(* Logix 5000 AddOnInstructionDefinition export Banner_IC70_Param_v4; software revision 33.03; part 2 of 2 *)
(* tags used below, declared in another part *)
   Hub : Banner_IC70_16P_v4;
   Port_Data : Banner_IOL_Port_v4;
   Port : INT;
   Control : DINT;
   Command_Being_Processed : BOOL;
   Index_Write_Inprocess : INT;
   Inprocess_Index : DINT;
   Index5 : SINT;
(* Banner_IC70_Param_v4, continued *)

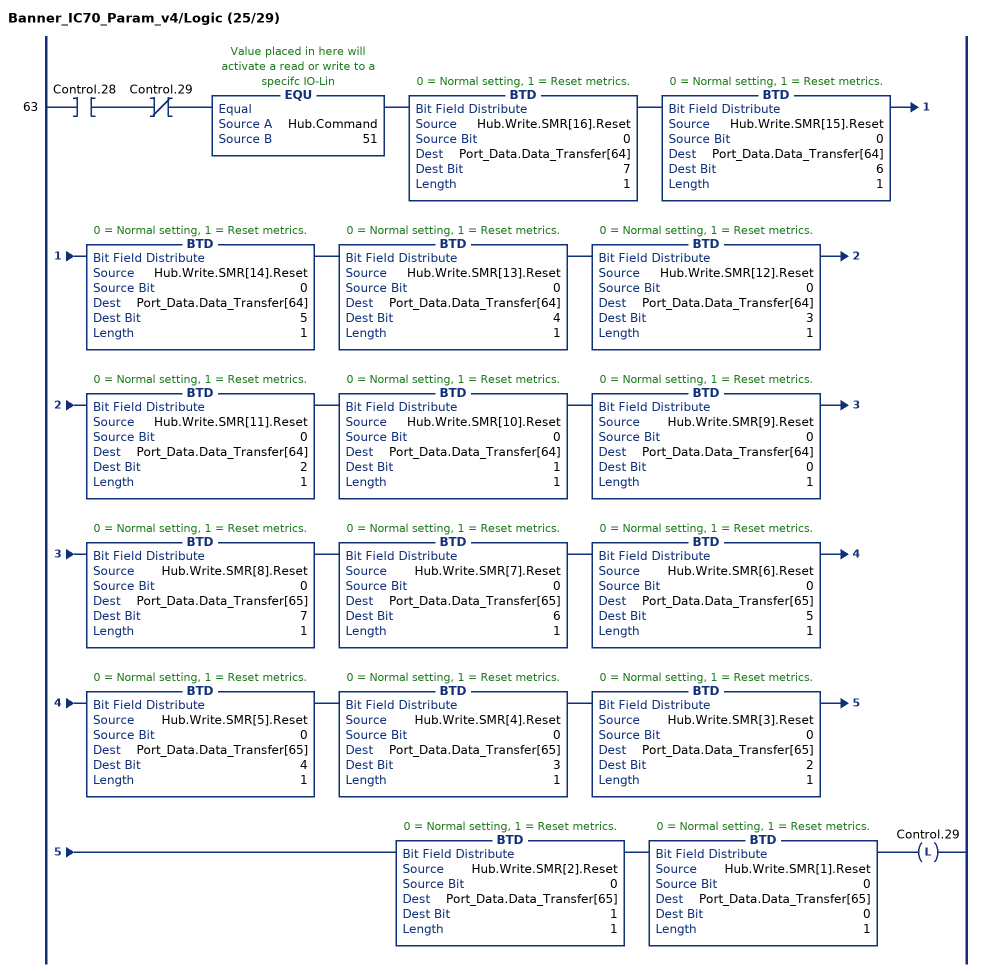
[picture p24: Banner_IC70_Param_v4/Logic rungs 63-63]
   63: XIC(Control.28)XIO(Control.29)EQU(Hub.Command,51)BTD(Hub.Write.SMR[16].Reset,0,Port_Data.Data_Transfer[64],7,1)BTD(Hub.Write.SMR[15].Reset,0,Port_Data.Data_Transfer[64],6,1)BTD(Hub.Write.SMR[14].Reset,0,Port_Data.Data_Transfer[64],5,1)BTD(Hub.Write.SMR[13].Reset,0,Port_Data.Data_Transfer[64],4,1)BTD(Hub.Write.SMR[12].Reset,0,Port_Data.Data_Transfer[64],3,1)BTD(Hub.Write.SMR[11].Reset,0,Port_Data.Data_Transfer[64],2,1)BTD(Hub.Write.SMR[10].Reset,0,Port_Data.Data_Transfer[64],1,1)BTD(Hub.Write.SMR[9].Reset,0,Port_Data.Data_Transfer[64],0,1)BTD(Hub.Write.SMR[8].Reset,0,Port_Data.Data_Transfer[65],7,1)BTD(Hub.Write.SMR[7].Reset,0,Port_Data.Data_Transfer[65],6,1)BTD(Hub.Write.SMR[6].Reset,0,Port_Data.Data_Transfer[65],5,1)BTD(Hub.Write.SMR[5].Reset,0,Port_Data.Data_Transfer[65],4,1)BTD(Hub.Write.SMR[4].Reset,0,Port_Data.Data_Transfer[65],3,1)BTD(Hub.Write.SMR[3].Reset,0,Port_Data.Data_Transfer[65],2,1)BTD(Hub.Write.SMR[2].Reset,0,Port_Data.Data_Transfer[65],1,1)BTD(Hub.Write.SMR[1].Reset,0,Port_Data.Data_Transfer[65],0,1)OTL(Control.29);
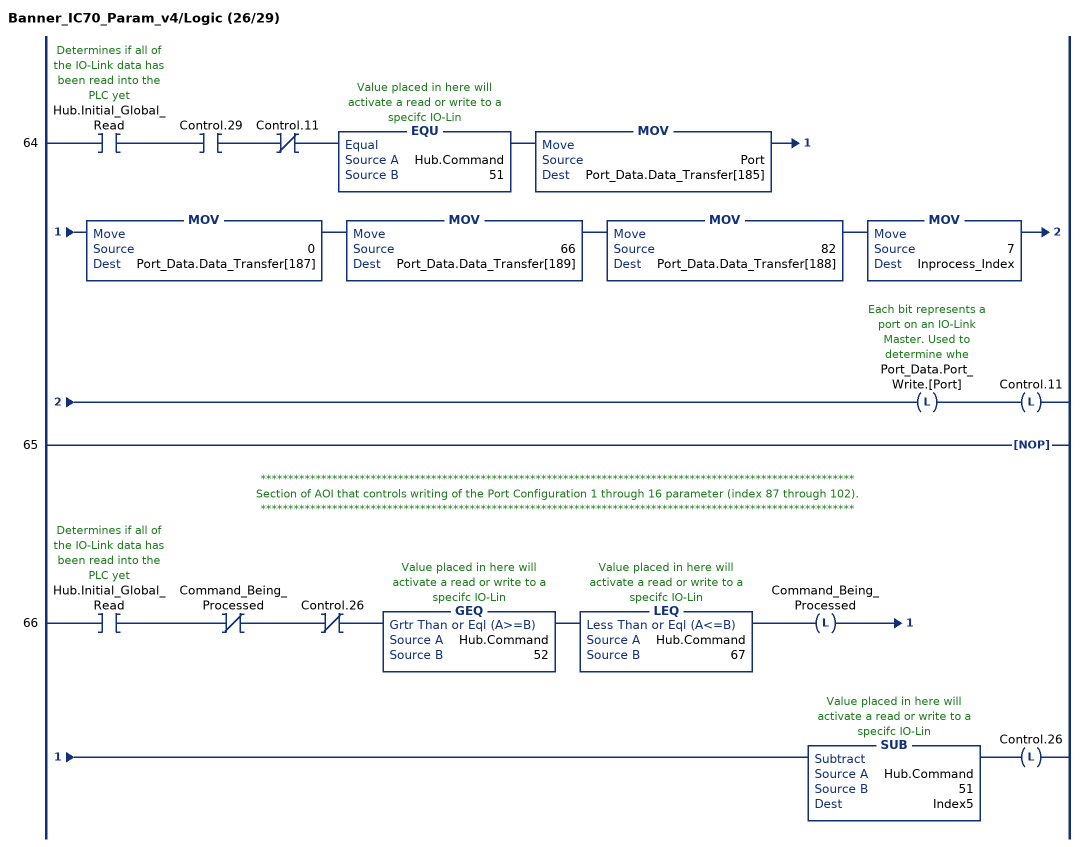
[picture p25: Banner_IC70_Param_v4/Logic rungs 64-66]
   64: XIC(Hub.Initial_Global_Read)XIC(Control.29)XIO(Control.11)EQU(Hub.Command,51)MOV(Port,Port_Data.Data_Transfer[185])MOV(0,Port_Data.Data_Transfer[187])MOV(66,Port_Data.Data_Transfer[189])MOV(82,Port_Data.Data_Transfer[188])MOV(7,Inprocess_Index)OTL(Port_Data.Port_Write.[Port])OTL(Control.11);
   65: NOP();
   // ************************************************************************************************************
   // Section of AOI that controls writing of the Port Configuration 1 through 16 parameter (index 87 through 102).
   // ************************************************************************************************************
   66: XIC(Hub.Initial_Global_Read)XIO(Command_Being_Processed)XIO(Control.26)GEQ(Hub.Command,52)LEQ(Hub.Command,67)OTL(Command_Being_Processed)SUB(Hub.Command,51,Index5)OTL(Control.26);
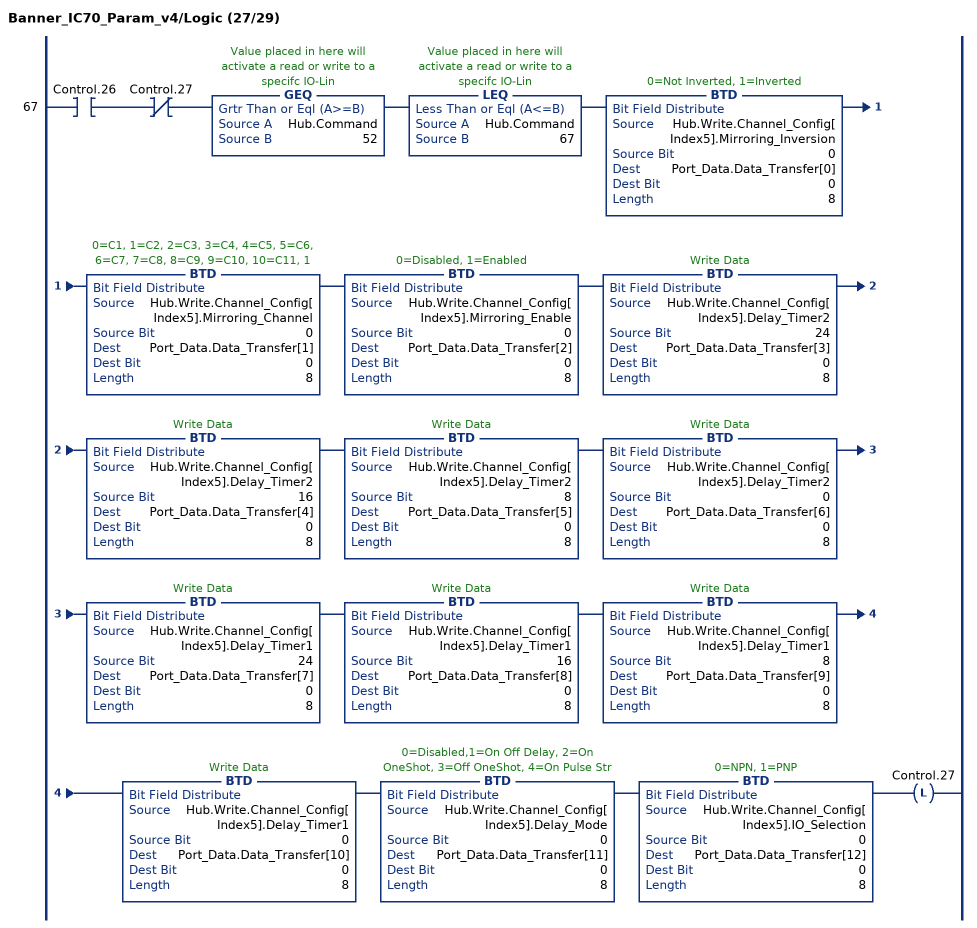
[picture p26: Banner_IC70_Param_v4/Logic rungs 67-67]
   67: XIC(Control.26)XIO(Control.27)GEQ(Hub.Command,52)LEQ(Hub.Command,67)BTD(Hub.Write.Channel_Config[Index5].Mirroring_Inversion,0,Port_Data.Data_Transfer[0],0,8)BTD(Hub.Write.Channel_Config[Index5].Mirroring_Channel,0,Port_Data.Data_Transfer[1],0,8)BTD(Hub.Write.Channel_Config[Index5].Mirroring_Enable,0,Port_Data.Data_Transfer[2],0,8)BTD(Hub.Write.Channel_Config[Index5].Delay_Timer2,24,Port_Data.Data_Transfer[3],0,8)BTD(Hub.Write.Channel_Config[Index5].Delay_Timer2,16,Port_Data.Data_Transfer[4],0,8)BTD(Hub.Write.Channel_Config[Index5].Delay_Timer2,8,Port_Data.Data_Transfer[5],0,8)BTD(Hub.Write.Channel_Config[Index5].Delay_Timer2,0,Port_Data.Data_Transfer[6],0,8)BTD(Hub.Write.Channel_Config[Index5].Delay_Timer1,24,Port_Data.Data_Transfer[7],0,8)BTD(Hub.Write.Channel_Config[Index5].Delay_Timer1,16,Port_Data.Data_Transfer[8],0,8)BTD(Hub.Write.Channel_Config[Index5].Delay_Timer1,8,Port_Data.Data_Transfer[9],0,8)BTD(Hub.Write.Channel_Config[Index5].Delay_Timer1,0,Port_Data.Data_Transfer[10],0,8)BTD(Hub.Write.Channel_Config[Index5].Delay_Mode,0,Port_Data.Data_Transfer[11],0,8)BTD(Hub.Write.Channel_Config[Index5].IO_Selection,0,Port_Data.Data_Transfer[12],0,8)OTL(Control.27);
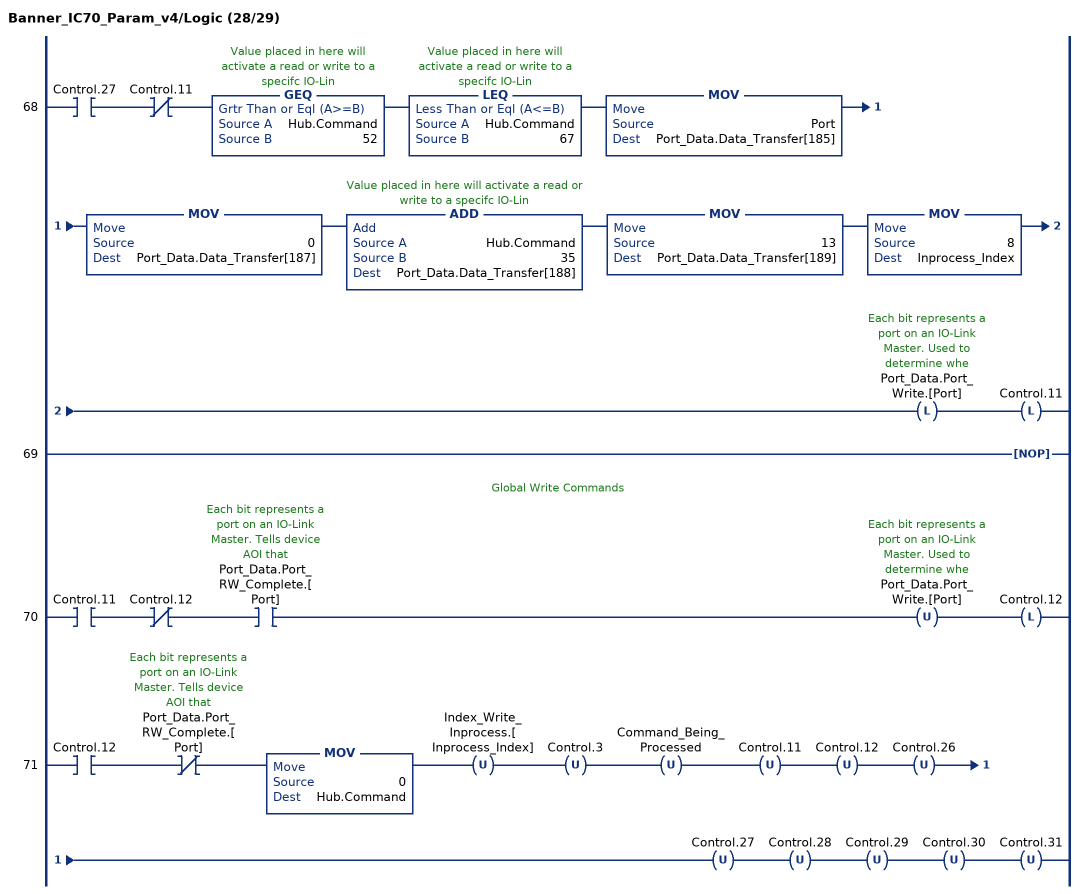
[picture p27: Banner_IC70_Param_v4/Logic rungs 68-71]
   68: XIC(Control.27)XIO(Control.11)GEQ(Hub.Command,52)LEQ(Hub.Command,67)MOV(Port,Port_Data.Data_Transfer[185])MOV(0,Port_Data.Data_Transfer[187])ADD(Hub.Command,35,Port_Data.Data_Transfer[188])MOV(13,Port_Data.Data_Transfer[189])MOV(8,Inprocess_Index)OTL(Port_Data.Port_Write.[Port])OTL(Control.11);
   69: NOP();
   // Global Write Commands
   70: XIC(Control.11)XIO(Control.12)XIC(Port_Data.Port_RW_Complete.[Port])OTU(Port_Data.Port_Write.[Port])OTL(Control.12);
   71: XIC(Control.12)XIO(Port_Data.Port_RW_Complete.[Port])MOV(0,Hub.Command)OTU(Index_Write_Inprocess.[Inprocess_Index])OTU(Control.3)OTU(Command_Being_Processed)OTU(Control.11)OTU(Control.12)OTU(Control.26)OTU(Control.27)OTU(Control.28)OTU(Control.29)OTU(Control.30)OTU(Control.31);
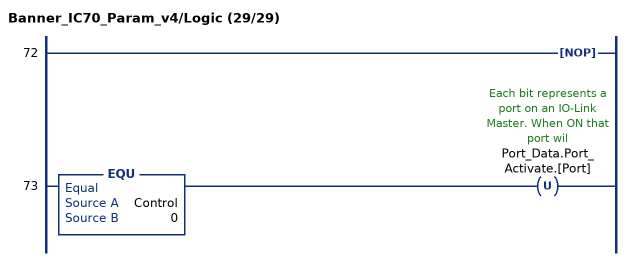
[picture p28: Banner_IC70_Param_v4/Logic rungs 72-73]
   72: NOP();
   73: EQU(Control,0)OTU(Port_Data.Port_Activate.[Port]);
END_ROUTINE
END_ADD_ON_INSTRUCTION
